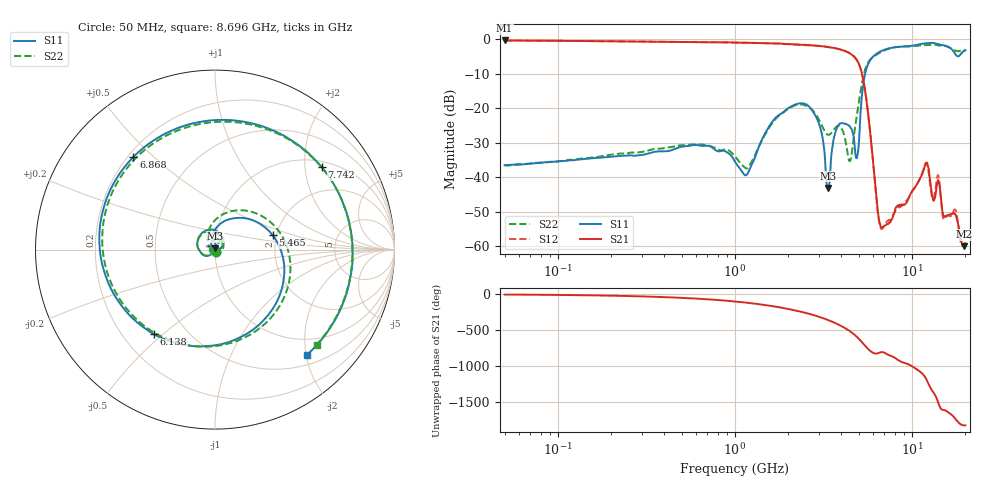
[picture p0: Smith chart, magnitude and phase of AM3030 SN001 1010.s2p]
# Hz S DB R 50
!freq MagS11 AngS11 MagS21 AngS21 MagS12 AngS12 MagS22 AngS22
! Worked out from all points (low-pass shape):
!   1601 points, 50 MHz to 20.05 GHz, reference 50 ohm
!   highest |S21| = -0.39 dB at 50 MHz (marker M1); lowest = -59.9 dB at 19.6 GHz (marker M2)
!   |S21| within 3 dB of the highest: start of sweep to 4.163 GHz
!   lowest |S11| = -43.1 dB at 3.358 GHz (marker M3), VSWR 1.01, Z = 50.2 + j0.661 ohm
!   |S11| at or under -10 dB: start of sweep to 5.441 GHz
!   |S22| runs from -37.5 to -1.6 dB; largest |S21 - S12| = 0.014
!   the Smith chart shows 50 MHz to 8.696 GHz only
!   S11 on the Smith chart (normalised r, x): 50 MHz: 1.01, -0.03; 5.465 GHz: 1.91, +0.34; 6.138 GHz: 0.33, -0.47; 6.868 GHz: 0.22, +0.43; 7.742 GHz: 1.16, +2.45; 8.696 GHz: 0.67, -2.01
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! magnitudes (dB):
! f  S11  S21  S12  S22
! 50 MHz  -36.5  -0.4  -0.4  -36.5
! 135.9 MHz  -34.8  -0.6  -0.6  -34.6
! 369.6 MHz  -32.5  -0.8  -0.8  -31.7
! 1.005 GHz  -35.6  -1.0  -1.0  -34.0
! 1.163 GHz  -39.3  -1.1  -1.1  -37.4
! 1.704 GHz  -22.7  -1.3  -1.2  -23.0
! 2.722 GHz  -20.5  -1.8  -1.9  -20.4
! 3.069 GHz  -26.6  -2.1  -2.0  -24.6
! 3.358 GHz  -43.1  -2.3  -2.3  -27.7
! 3.757 GHz  -25.9  -2.7  -2.7  -25.3
! 4.481 GHz  -25.4  -4.2  -4.2  -35.2
! 4.902 GHz  -34.2  -6.2  -6.2  -21.5
! 5.465 GHz  -9.6  -15.6  -15.6  -8.5
! 6.138 GHz  -4.7  -39.8  -39.9  -4.9
! 6.868 GHz  -3.3  -54.4  -54.6  -3.5
! 7.402 GHz  -2.7  -53.3  -52.5  -2.8
! 7.742 GHz  -2.5  -52.0  -51.4  -2.5
! 8.696 GHz  -2.2  -48.3  -48.4  -2.2
! 12 GHz  -1.2  -35.9  -35.8  -1.8
! 13.03 GHz  -1.1  -45.5  -46.0  -1.6
! 19.6 GHz  -3.5  -59.9  -59.6  -3.2
! 20.05 GHz  -3.3  -59.2  -59.0  -3.2
